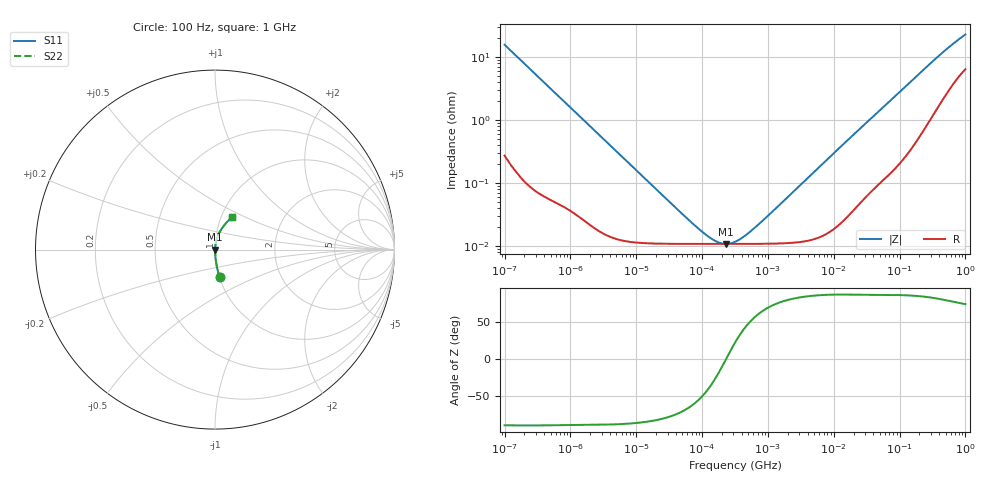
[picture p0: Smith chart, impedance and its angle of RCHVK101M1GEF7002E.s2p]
! RCHVK101M1GEF7002E  S-PARAMETER MODEL  (AEC-Q200 qualified)
! Model Generated by ELNA Corporation (http://www.ty-top.com)
! Version 1.0
! ELNA Control No. 240315
! Copyright (c) 2024 ELNA CO.,LTD. All Rights Reserved.
! Products Name : CONDUCTIVE POLYMER HYBRID ALUMINUM ELECTROLYTIC CAPACITORS
! Characteristics :
!  Capacitance  :  100uF  ,  Rated voltage  :  35V
!  Operating Temp. Range  :  -55 to +125 degC  ,  Endurance  :  4000hr at 125 degC
!  Dimension D  :  8mm  ,  Dimension L  :  8.7mm
! Frequency Range : 100Hz - 1GHz
! External Node Assignments :
!  1  o---| |---o  2
# MHz S RI R 50
!Freq[MHz].  S11 Real  S11 Imag  S21 Real  S21 Imag  S12 Real  S12 Imag  S22 Real  S22 Imag
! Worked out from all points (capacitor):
!   401 points, 100 Hz to 1 GHz, reference 50 ohm
!   read as one part in series: C = 102 uF near 108 Hz
!   lowest |Z| = 10.9 mohm at 229.1 kHz (marker M1)
!   series resonance near 231.7 kHz, so ESL is about 4.6 nH
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0.0001  0.0261 -0.151  0.9739 0.151  0.9739 0.151  0.0261 -0.151
0.000113  0.0207 -0.1346  0.9793 0.1346  0.9793 0.1346  0.0207 -0.1346
0.000183  0.00831 -0.0842  0.9917 0.0842  0.9917 0.0842  0.00831 -0.0842
0.000309  0.00325 -0.0502  0.9968 0.0502  0.9968 0.0502  0.00325 -0.0502
0.001488  0.000384 -0.0106  0.9996 0.0106  0.9996 0.0106  0.000384 -0.0106
0.022131  0.00011 -0.000717  0.9999 0.000717  0.9999 0.000717  0.00011 -0.000717
0.063096  0.000109 -0.000235  0.9999 0.000235  0.9999 0.000235  0.000109 -0.000235
0.110917  0.000109 -0.000111  0.9999 0.000111  0.9999 0.000111  0.000109 -0.000111
0.165959  0.000109 -4.69e-05  0.9999 4.69e-05  0.9999 4.69e-05  0.000109 -4.69e-05
0.194984  0.000109 -2.39e-05  0.9999 2.39e-05  0.9999 2.39e-05  0.000109 -2.39e-05
0.229087  0.000109 -1.53e-06  0.9999 1.53e-06  0.9999 1.53e-06  0.000109 -1.53e-06
0.269153  0.000109 2.08e-05  0.9999 -2.08e-05  0.9999 -2.08e-05  0.000109 2.08e-05
0.316228  0.000109 4.37e-05  0.9999 -4.37e-05  0.9999 -4.37e-05  0.000109 4.37e-05
0.436516  0.000109 9.36e-05  0.9999 -9.36e-05  0.9999 -9.36e-05  0.000109 9.36e-05
0.653131  0.000109 0.00017  0.9999 -0.00017  0.9999 -0.00017  0.000109 0.00017
4.704354  0.000129 0.0014  0.9999 -0.0014  0.9999 -0.0014  0.000129 0.0014
17.08048  0.000336 0.00501  0.9997 -0.00501  0.9997 -0.00501  0.000336 0.00501
69.9842  0.00175 0.0194  0.9983 -0.0194  0.9983 -0.0194  0.00175 0.0194
176.8072  0.00666 0.0474  0.9933 -0.0474  0.9933 -0.0474  0.00666 0.0474
395.8221  0.0264 0.0982  0.9736 -0.0982  0.9736 -0.0982  0.0264 0.0982
668.3439  0.0592 0.1452  0.9408 -0.1452  0.9408 -0.1452  0.0592 0.1452
1000  0.0974 0.184  0.9026 -0.184  0.9026 -0.184  0.0974 0.184
